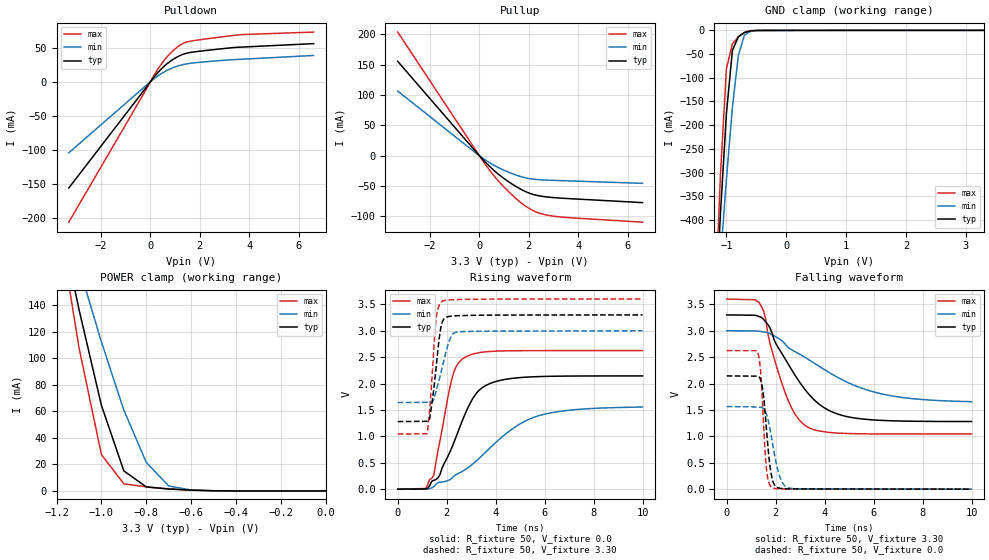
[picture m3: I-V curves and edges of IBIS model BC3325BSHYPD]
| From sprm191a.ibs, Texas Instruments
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[Model]   BC3325BSHYPD
Model_type   I/O
Vinh = 2.00
Vinl = 0.80
Enable   Active-Low
Polarity   Non-Inverting
| signals   A, GZ, Y
Vmeas = 1.5
|   typ   min   max
C_comp   1.4592p   1.4336p   1.5063p
|   typ   min   max
[Temperature Range]   25   -40   125
|   typ   min   max
[Voltage Range]   3.30V   3.00V   3.60V
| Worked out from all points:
|   slope of the pulldown table from 0 to 0.495 V, typ, clamps not added: 24 ohm
|   slope of the pullup table from 0 to 0.495 V, typ, clamps not added: 23.8 ohm
|   GND clamp passes 1 mA (typ) near -0.60 V on its own axis
|   POWER clamp passes 1 mA (typ) near -0.65 V on its own axis
|   rising waveform, R_fixture 50, V_fixture 0.0: 20-80 % time 1.22ns typ, 2.5ns min, 650ps max; typ from 0 V to 2.15 V
|   falling waveform, R_fixture 50, V_fixture 3.30: 20-80 % time 1.7ns typ, 3.02ns min, 999ps max; typ from 3.3 V to 1.28 V
|   rising waveform, R_fixture 50, V_fixture 3.30: 20-80 % time 294ps typ, 451ps min, 227ps max; typ from 1.28 V to 3.3 V
|   falling waveform, R_fixture 50, V_fixture 0.0: 20-80 % time 254ps typ, 399ps min, 190ps max; typ from 2.15 V to 0 V
[Pulldown]
|   Voltage   I(typ)   I(min)   I(max)
-3.3V     -155.5mA   -104mA     -205.5mA
200mV     9.24mA     5.864mA    12.69mA
600mV     24.12mA    15.27mA    33.29mA
800mV     29.86mA    18.87mA    41.36mA
1.1V      36.62mA    23.02mA    51.07mA
1.3V      39.96mA    25.04mA    55.82mA
1.6V      42.83mA    27mA       59.29mA
3.5V      50.44mA    32.65mA    68.4mA
6.6V      55.85mA    38.51mA    72.75mA
[GND_clamp]
|   Voltage   I(typ)   I(min)   I(max)
-3.3V     -6.297A    -4.744A    -8.187A
-1.2V     -628.7mA   -661.8mA   -615.9mA
-1.1V     -388.2mA   -483.6mA   -305.7mA
-1V       -175.3mA   -314.3mA   -80.82mA
-900mV    -42.2mA    -162.8mA   -28.51mA
-800mV    -13.03mA   -52.28mA   -13.66mA
-700mV    -4.731mA   -10.22mA   -4.038mA
-600mV    -956.9uA   -2.319mA   -531.6uA
-400mV    -40.57uA   -70.41uA   -55.7uA
3.3V      100.3uA    53.84uA    176.6uA
[Pullup]
|   Voltage   I(typ)   I(min)   I(max)
-3.3V     155.5mA    106.5mA    203.9mA
-200mV    9.306mA    6.232mA    12.42mA
300mV     -13.07mA   -8.546mA   -17.75mA
600mV     -24.68mA   -16mA      -33.65mA
900mV     -34.78mA   -22.33mA   -47.64mA
1.4V      -48.81mA   -30.79mA   -67.77mA
1.7V      -55.9mA    -34.78mA   -78.19mA
2V        -61.53mA   -37.68mA   -86.7mA
2.3V      -65.32mA   -39.23mA   -93.02mA
2.9V      -68.85mA   -40.62mA   -99.23mA
3.7V      -71.04mA   -41.74mA   -102.5mA
6.6V      -77.5mA    -45.68mA   -109.8mA
[POWER_clamp]
|   Voltage   I(typ)   I(min)   I(max)
-3.3V     2.11A      1.592A     2.74A
-1.2V     217.5mA    228.7mA    212.8mA
-1.1V     136.8mA    169mA      108.1mA
-1V       64.49mA    112.2mA    27.39mA
-900mV    15.08mA    60.9mA     5.337mA
-800mV    3.01mA     21.46mA    3.051mA
-700mV    1.426mA    3.716mA    1.578mA
-600mV    596.1uA    671uA      553.1uA
0V        0A         0A         0A
[Ramp]
|   I(typ)   I(min)   I(max)
dV/dt_r   1.287/1.225n   0.933/2.497n   1.574/0.650n
dV/dt_f   1.212/1.701n   0.806/3.021n   1.534/1.000n
[Rising Waveform]
R_fixture = 50
V_fixture = 0.0
|  pu_on
|  TIME   V(typ)   V(min)   V(max)
0s        3nV        16nV       2nV
1.143ns   3.636mV    53.19uV    12.63mV
1.476ns   168mV      48.56mV    269.7mV
1.726ns   278.3mV    130.1mV    920.6mV
2.226ns   805.3mV    213mV      2.115V
2.726ns   1.395V     362.2mV    2.491V
3.142ns   1.769V     507.9mV    2.568V
3.559ns   1.953V     687mV      2.599V
5.558ns   2.128V     1.36V      2.623V
10ns      2.145V     1.555V     2.624V
[Falling Waveform]
R_fixture = 50
V_fixture = 3.30
V_fixture_min = 3.00
V_fixture_max = 3.60
|  pd_on
|  TIME   V(typ)   V(min)   V(max)
0s        3.3V       3V         3.6V
1.327ns   3.268V     2.99V      3.534V
1.502ns   3.218V     2.977V     3.38V
1.85ns    2.957V     2.927V     2.624V
2.461ns   2.41V      2.707V     1.739V
2.81ns    2.145V     2.6V       1.408V
3.333ns   1.81V      2.458V     1.171V
5.077ns   1.359V     1.993V     1.052V
7.083ns   1.291V     1.742V     1.044V
10ns      1.281V     1.657V     1.044V
[Rising Waveform]
R_fixture = 50
V_fixture = 3.30
V_fixture_min = 3.00
V_fixture_max = 3.60
|  pd_off
|  TIME   V(typ)   V(min)   V(max)
0s        1.28V      1.641V     1.044V
1.192ns   1.285V     1.645V     1.05V
1.304ns   1.339V     1.651V     1.516V
1.444ns   1.792V     1.673V     2.439V
1.556ns   2.253V     1.841V     3.181V
1.697ns   2.86V      2.08V      3.487V
1.809ns   3.151V     2.288V     3.556V
2.117ns   3.272V     2.822V     3.583V
2.397ns   3.284V     2.973V     3.59V
10ns      3.3V       3V         3.6V
[Falling Waveform]
R_fixture = 50
V_fixture = 0.0
|  pu_off
|  TIME   V(typ)   V(min)   V(max)
0s        2.145V     1.565V     2.624V
1.277ns   2.141V     1.551V     2.576V
1.402ns   2.04V      1.551V     2.144V
1.509ns   1.754V     1.522V     1.206V
1.634ns   1.083V     1.405V     348.1mV
1.759ns   472.8mV    1.166V     85.66mV
1.866ns   182.8mV    888.3mV    27.6mV
2.187ns   16.3mV     215.7mV    6.863mV
2.527ns   6.442mV    24.49mV    3.663mV
10ns      2.369uV    60.69uV    374.4nV
